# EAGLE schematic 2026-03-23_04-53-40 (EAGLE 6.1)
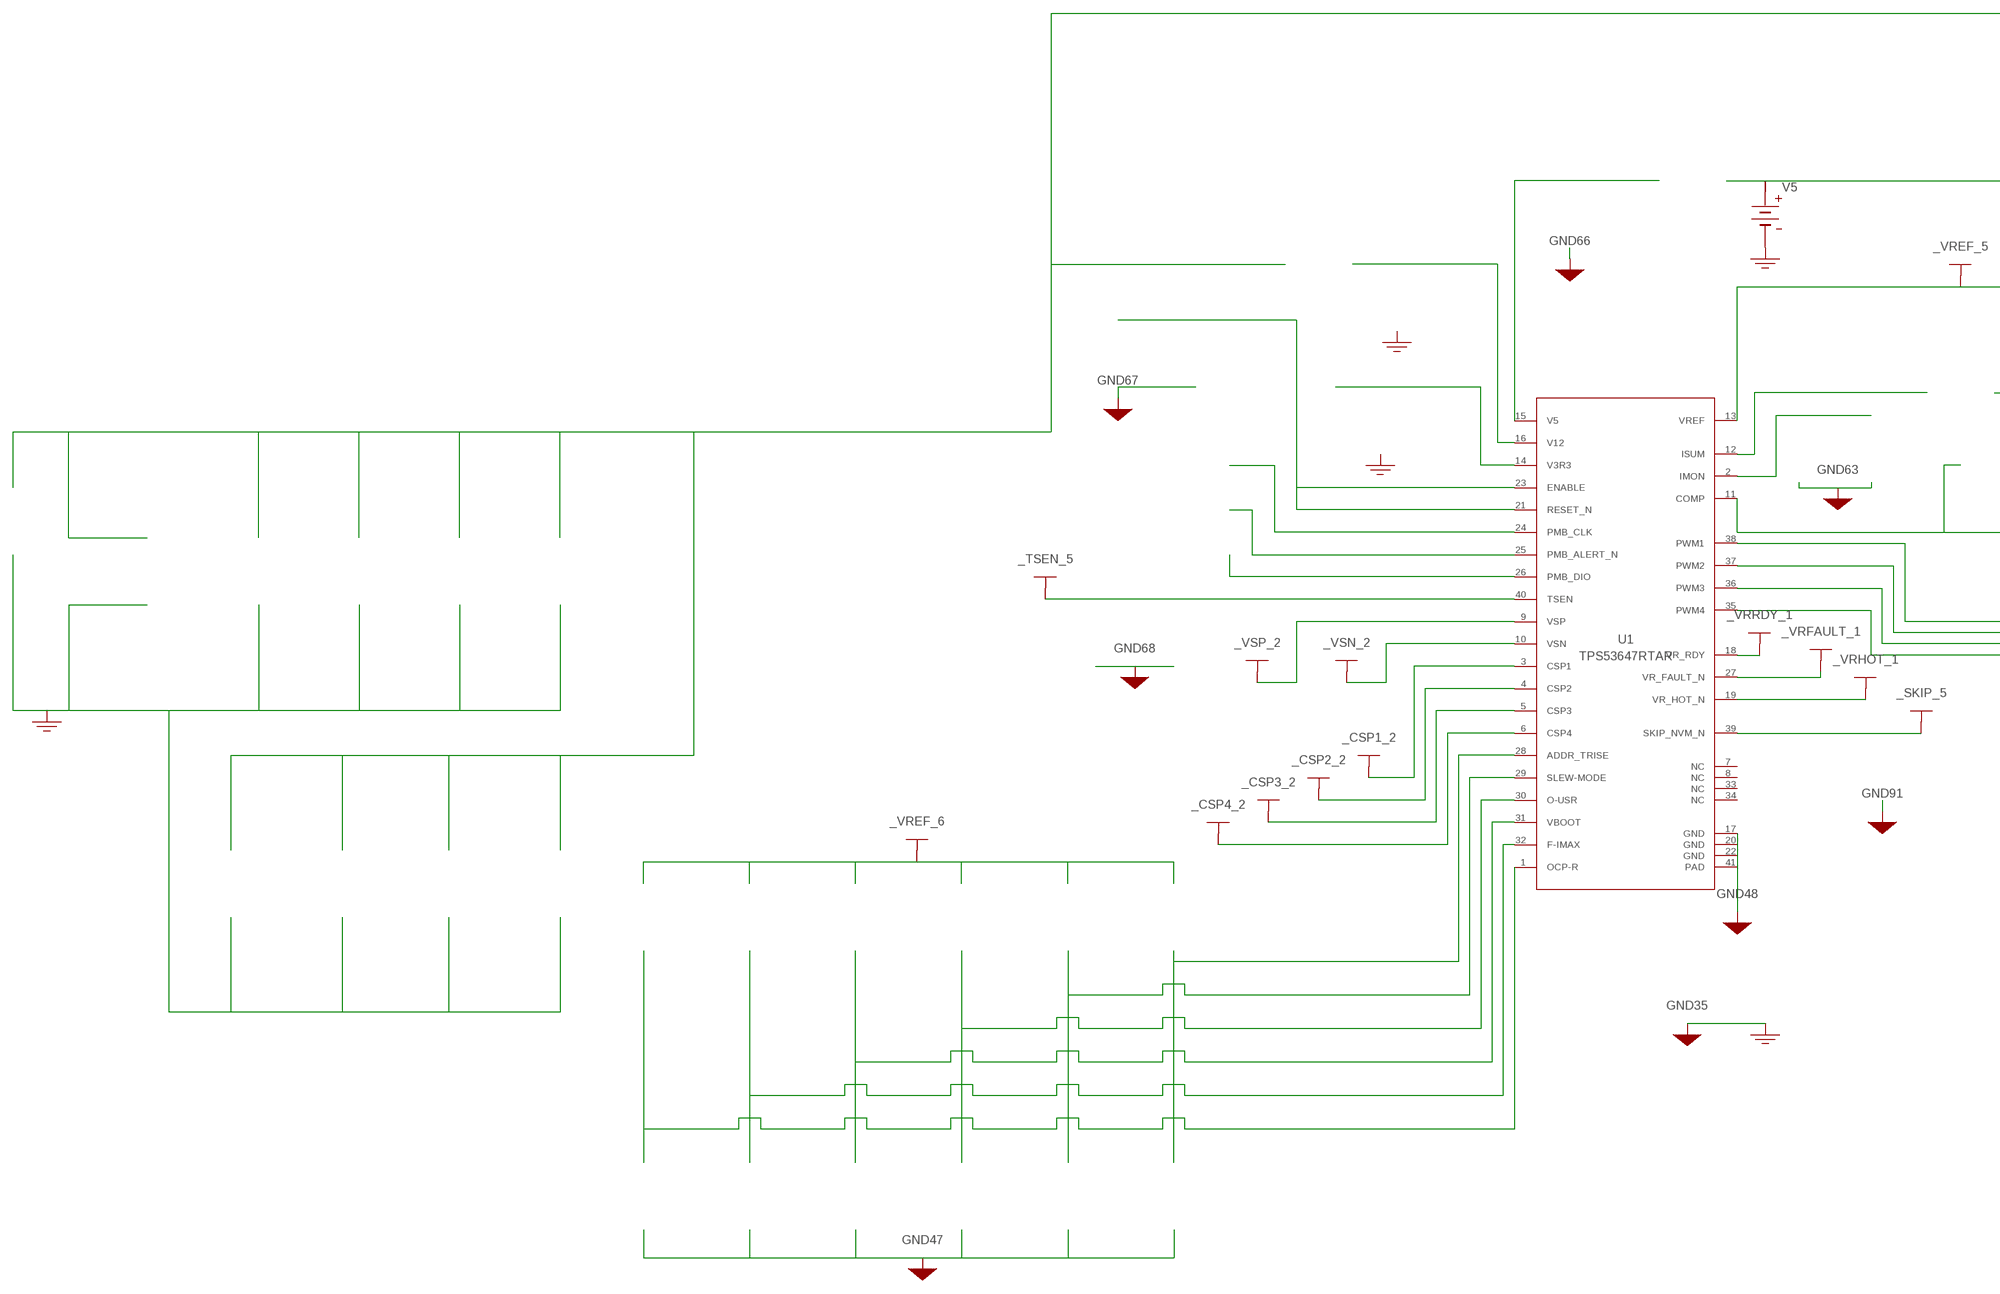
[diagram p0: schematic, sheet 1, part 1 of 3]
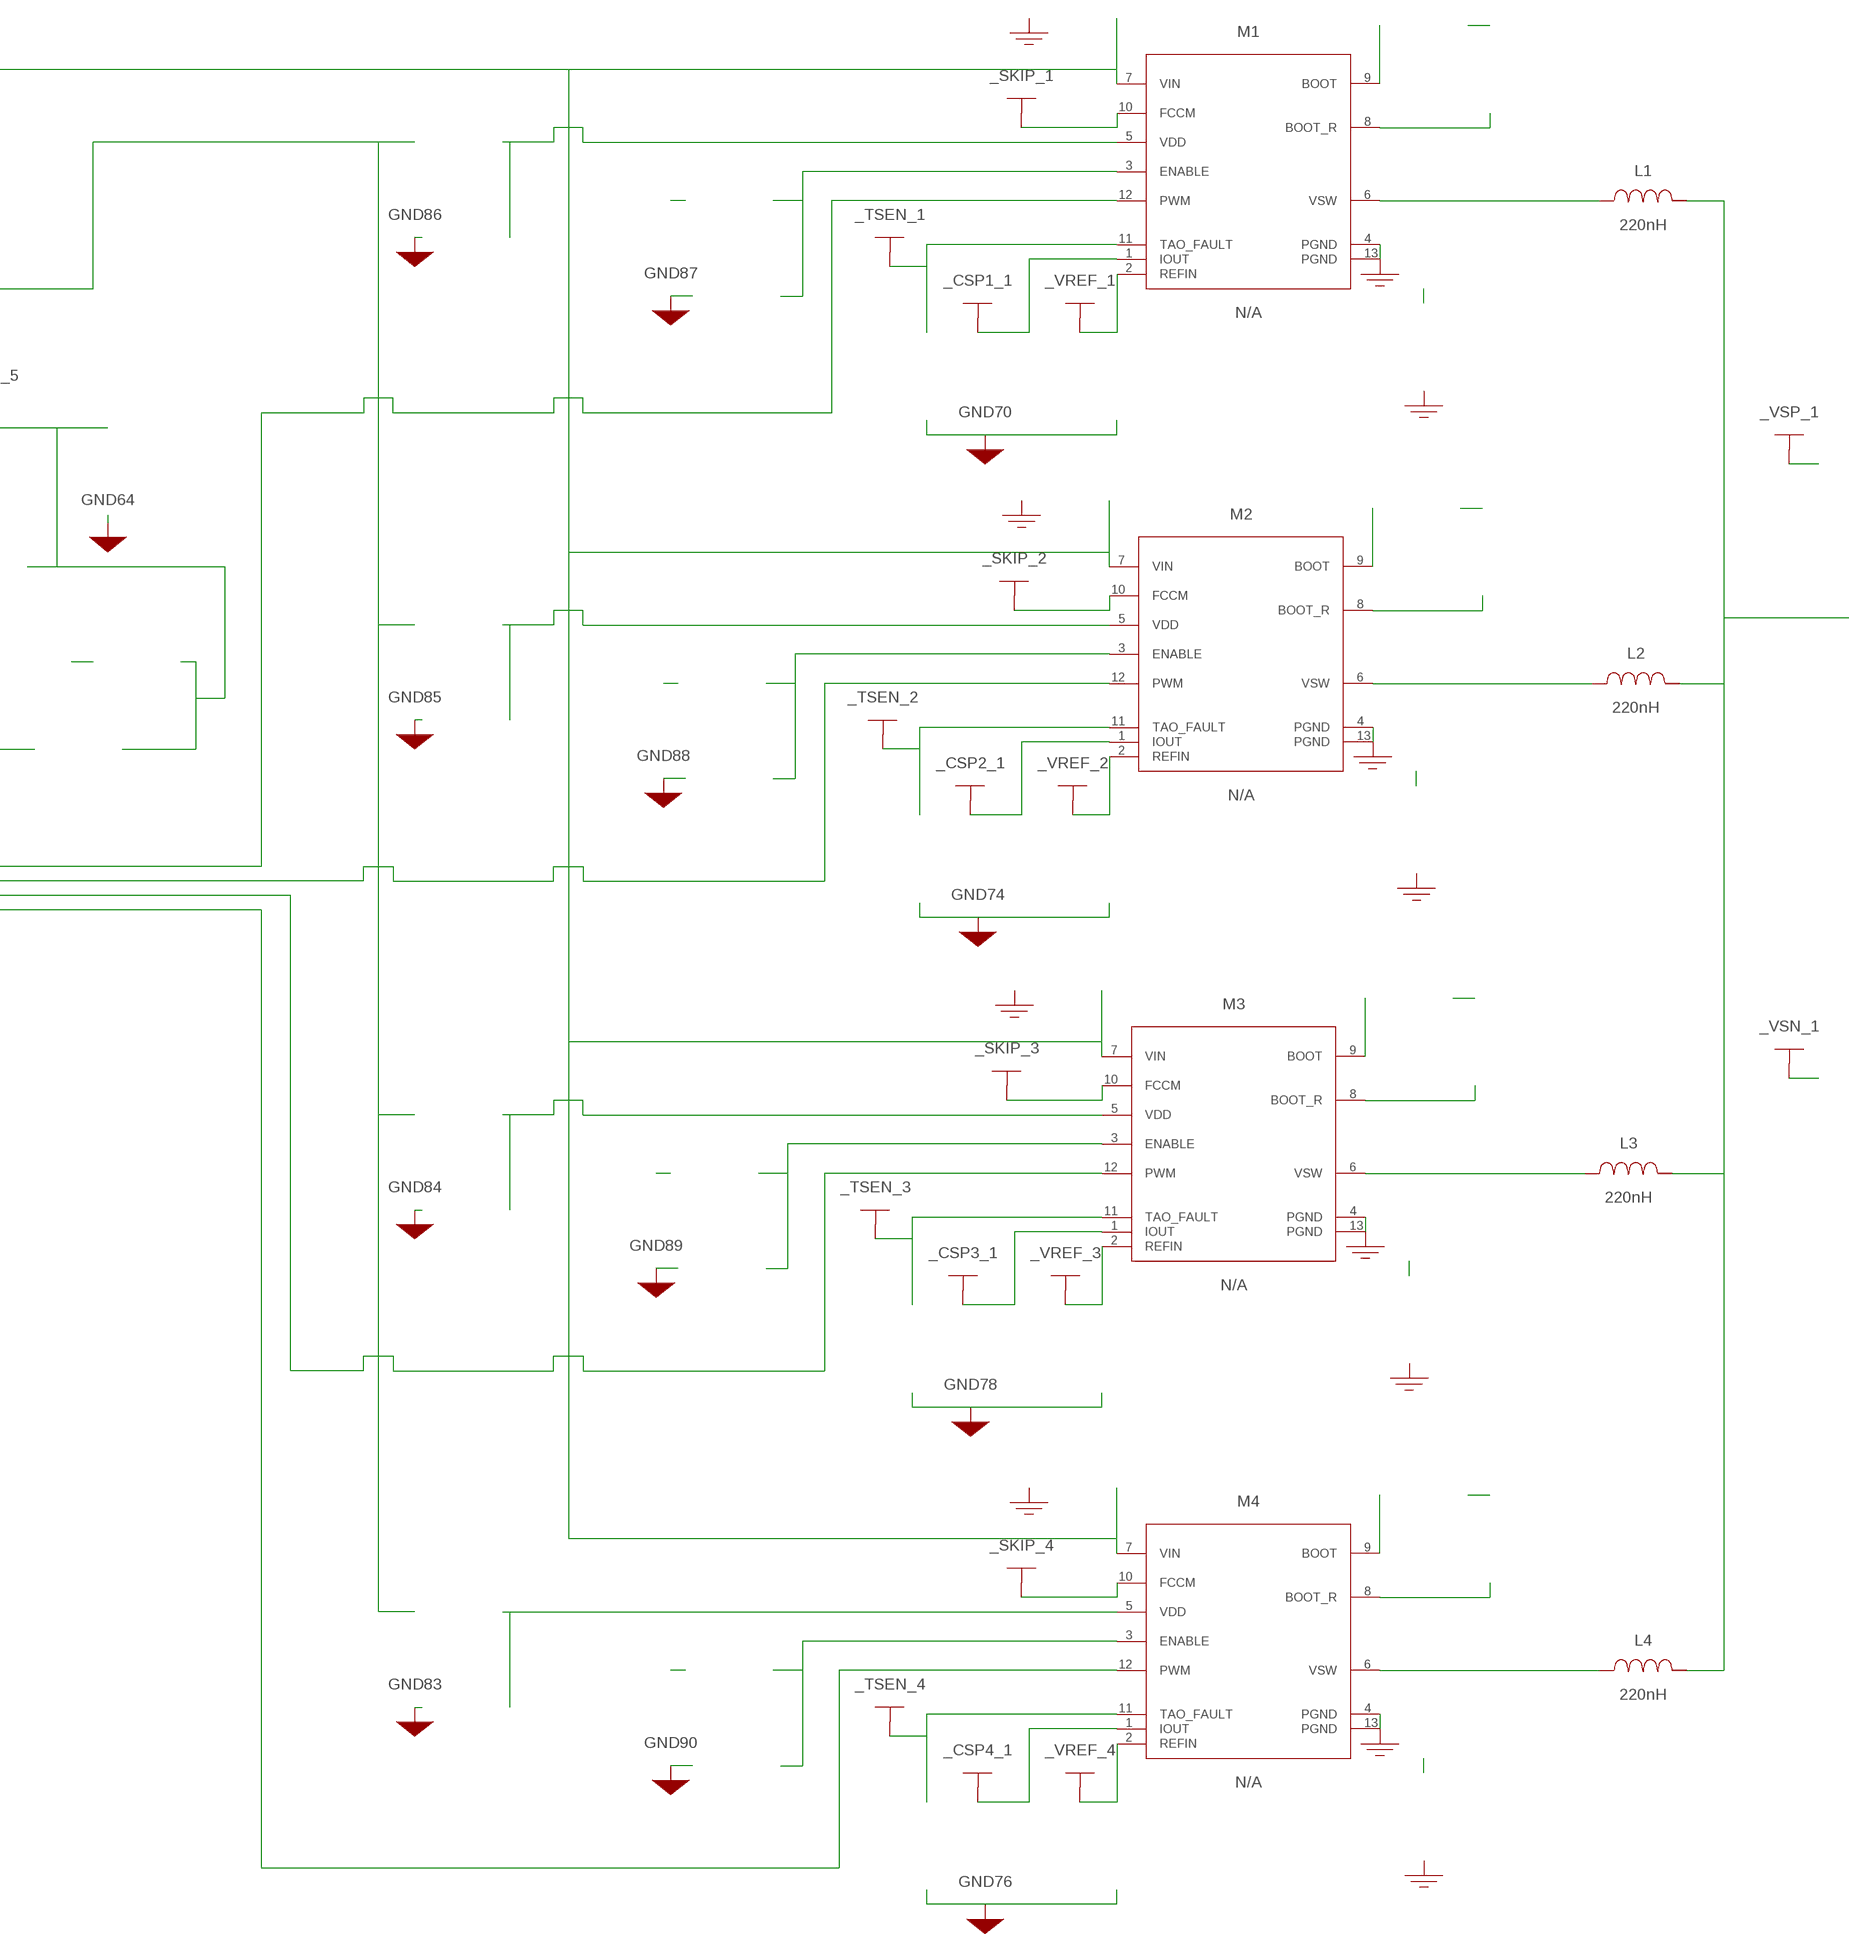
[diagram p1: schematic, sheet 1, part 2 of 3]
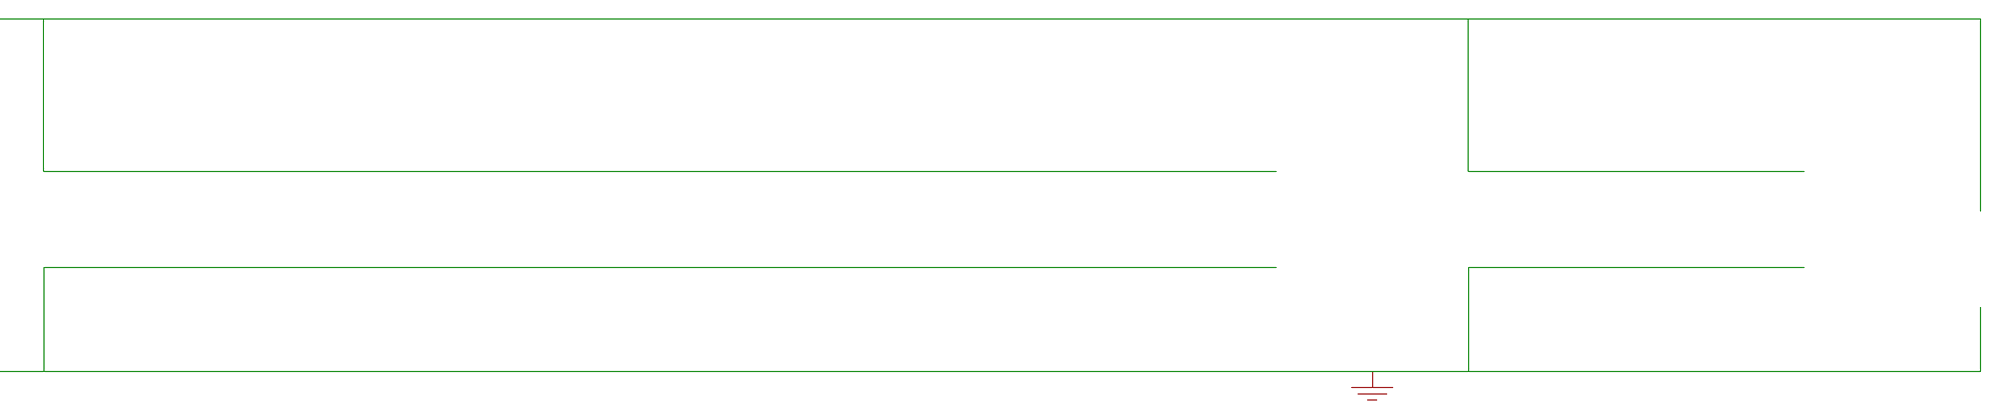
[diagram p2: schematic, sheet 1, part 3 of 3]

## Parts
_CSP1_1  WB_CONTINUATION  WB_CONTINUATIONWB_CONTINUATION  [WB_CONTINUATION]
_CSP1_2  WB_CONTINUATION  WB_CONTINUATIONWB_CONTINUATION  [WB_CONTINUATION]
_CSP2_1  WB_CONTINUATION  WB_CONTINUATIONWB_CONTINUATION  [WB_CONTINUATION]
_CSP2_2  WB_CONTINUATION  WB_CONTINUATIONWB_CONTINUATION  [WB_CONTINUATION]
_CSP3_1  WB_CONTINUATION  WB_CONTINUATIONWB_CONTINUATION  [WB_CONTINUATION]
_CSP3_2  WB_CONTINUATION  WB_CONTINUATIONWB_CONTINUATION  [WB_CONTINUATION]
_CSP4_1  WB_CONTINUATION  WB_CONTINUATIONWB_CONTINUATION  [WB_CONTINUATION]
_CSP4_2  WB_CONTINUATION  WB_CONTINUATIONWB_CONTINUATION  [WB_CONTINUATION]
_SKIP_1  WB_CONTINUATION  WB_CONTINUATIONWB_CONTINUATION  [WB_CONTINUATION]
_SKIP_2  WB_CONTINUATION  WB_CONTINUATIONWB_CONTINUATION  [WB_CONTINUATION]
_SKIP_3  WB_CONTINUATION  WB_CONTINUATIONWB_CONTINUATION  [WB_CONTINUATION]
_SKIP_4  WB_CONTINUATION  WB_CONTINUATIONWB_CONTINUATION  [WB_CONTINUATION]
_SKIP_5  WB_CONTINUATION  WB_CONTINUATIONWB_CONTINUATION  [WB_CONTINUATION]
_TSEN_1  WB_CONTINUATION  WB_CONTINUATIONWB_CONTINUATION  [WB_CONTINUATION]
_TSEN_2  WB_CONTINUATION  WB_CONTINUATIONWB_CONTINUATION  [WB_CONTINUATION]
_TSEN_3  WB_CONTINUATION  WB_CONTINUATIONWB_CONTINUATION  [WB_CONTINUATION]
_TSEN_4  WB_CONTINUATION  WB_CONTINUATIONWB_CONTINUATION  [WB_CONTINUATION]
_TSEN_5  WB_CONTINUATION  WB_CONTINUATIONWB_CONTINUATION  [WB_CONTINUATION]
_V3V3_1  WB_CONTINUATION  WB_CONTINUATIONWB_CONTINUATION  [WB_CONTINUATION]  (not placed on a sheet)
_V3V3_2  WB_CONTINUATION  WB_CONTINUATIONWB_CONTINUATION  [WB_CONTINUATION]  (not placed on a sheet)
_V3V3_3  WB_CONTINUATION  WB_CONTINUATIONWB_CONTINUATION  [WB_CONTINUATION]  (not placed on a sheet)
_V3V3_4  WB_CONTINUATION  WB_CONTINUATIONWB_CONTINUATION  [WB_CONTINUATION]  (not placed on a sheet)
_V3V3_5  WB_CONTINUATION  WB_CONTINUATIONWB_CONTINUATION  [WB_CONTINUATION]  (not placed on a sheet)
_VREF_1  WB_CONTINUATION  WB_CONTINUATIONWB_CONTINUATION  [WB_CONTINUATION]
_VREF_2  WB_CONTINUATION  WB_CONTINUATIONWB_CONTINUATION  [WB_CONTINUATION]
_VREF_3  WB_CONTINUATION  WB_CONTINUATIONWB_CONTINUATION  [WB_CONTINUATION]
_VREF_4  WB_CONTINUATION  WB_CONTINUATIONWB_CONTINUATION  [WB_CONTINUATION]
_VREF_5  WB_CONTINUATION  WB_CONTINUATIONWB_CONTINUATION  [WB_CONTINUATION]
_VREF_6  WB_CONTINUATION  WB_CONTINUATIONWB_CONTINUATION  [WB_CONTINUATION]
_VRFAULT_1  WB_CONTINUATION  WB_CONTINUATIONWB_CONTINUATION  [WB_CONTINUATION]
_VRHOT_1  WB_CONTINUATION  WB_CONTINUATIONWB_CONTINUATION  [WB_CONTINUATION]
_VRRDY_1  WB_CONTINUATION  WB_CONTINUATIONWB_CONTINUATION  [WB_CONTINUATION]
_VSN_1  WB_CONTINUATION  WB_CONTINUATIONWB_CONTINUATION  [WB_CONTINUATION]
_VSN_2  WB_CONTINUATION  WB_CONTINUATIONWB_CONTINUATION  [WB_CONTINUATION]
_VSP_1  WB_CONTINUATION  WB_CONTINUATIONWB_CONTINUATION  [WB_CONTINUATION]
_VSP_2  WB_CONTINUATION  WB_CONTINUATIONWB_CONTINUATION  [WB_CONTINUATION]
C3V3  1uF  C0603C105Z8VACTUC0603C105Z8VACTU  [0603]  (not placed on a sheet)
CBP3  1uF  C0603C105Z8VACTUC0603C105Z8VACTU  [0603]  (not placed on a sheet)
CBST1  100nF  EMK107B7104KA-TEMK107B7104KA-T  [0603]  (not placed on a sheet)
CBST2  100nF  EMK107B7104KA-TEMK107B7104KA-T  [0603]  (not placed on a sheet)
CBST3  100nF  EMK107B7104KA-TEMK107B7104KA-T  [0603]  (not placed on a sheet)
CBST4  100nF  EMK107B7104KA-TEMK107B7104KA-T  [0603]  (not placed on a sheet)
CCOMP  1nF  GRM1555C1H102JA01JGRM1555C1H102JA01J  [0402]  (not placed on a sheet)
CCOMP2  22pF  CL21C220JBANNNCCL21C220JBANNNC  [0805]  (not placed on a sheet)
CDD  1uF  C1608X5R1E105K080ACC1608X5R1E105K080AC  [0603]  (not placed on a sheet)
CEN1  1nF  CC0603JRNPO8BN102CC0603JRNPO8BN102  [0603]  (not placed on a sheet)
CEN2  1nF  CC0603JRNPO8BN102CC0603JRNPO8BN102  [0603]  (not placed on a sheet)
CEN3  1nF  CC0603JRNPO8BN102CC0603JRNPO8BN102  [0603]  (not placed on a sheet)
CEN4  1nF  CC0603JRNPO8BN102CC0603JRNPO8BN102  [0603]  (not placed on a sheet)
CHF1  3.3nF  CGA1A2X7R1E332K030BACGA1A2X7R1E332K030BA  [0201_033]  (not placed on a sheet)
CHF2  3.3nF  CGA1A2X7R1E332K030BACGA1A2X7R1E332K030BA  [0201_033]  (not placed on a sheet)
CHF3  3.3nF  CGA1A2X7R1E332K030BACGA1A2X7R1E332K030BA  [0201_033]  (not placed on a sheet)
CHF4  3.3nF  CGA1A2X7R1E332K030BACGA1A2X7R1E332K030BA  [0201_033]  (not placed on a sheet)
CIMON  2.2nF  GRM033R71A222KA01DGRM033R71A222KA01D  [0201]  (not placed on a sheet)
CIN  270uF  16SVPG270M16SVPG270M  [CAPSMT_62_C10]  (not placed on a sheet)
CIN_2  270uF  16SVPG270M16SVPG270M  [CAPSMT_62_C10]  (not placed on a sheet)
CINX_CH1  22uF  MSASE21GBB5226MTNA01MSASE21GBB5226MTNA01  [0805]  (not placed on a sheet)
CINX_CH2  22uF  MSASE21GBB5226MTNA01MSASE21GBB5226MTNA01  [0805]  (not placed on a sheet)
CINX_CH3  22uF  MSASE21GBB5226MTNA01MSASE21GBB5226MTNA01  [0805]  (not placed on a sheet)
CINX_CH4  22uF  MSASE21GBB5226MTNA01MSASE21GBB5226MTNA01  [0805]  (not placed on a sheet)
CINX_CH5  47uF  GRM32ER61C476KE15LGRM32ER61C476KE15L  [1210_280]  (not placed on a sheet)
CINX_CH6  47uF  GRM32ER61C476KE15LGRM32ER61C476KE15L  [1210_280]  (not placed on a sheet)
CINX_CH7  47uF  GRM32ER61C476KE15LGRM32ER61C476KE15L  [1210_280]  (not placed on a sheet)
CINX_CH8  47uF  GRM32ER61C476KE15LGRM32ER61C476KE15L  [1210_280]  (not placed on a sheet)
COUT  470uF  EEFGX0D471REEFGX0D471R  [7343-20]  (not placed on a sheet)
COUT_2  470uF  EEFGX0D471REEFGX0D471R  [7343-20]  (not placed on a sheet)
COUT_3  470uF  EEFGX0D471REEFGX0D471R  [7343-20]  (not placed on a sheet)
COUT_4  470uF  EEFGX0D471REEFGX0D471R  [7343-20]  (not placed on a sheet)
COUTX_CH1  100uF  GRM32EC80J107ME20LGRM32EC80J107ME20L  [1210_270]  (not placed on a sheet)
COUTX_CH1_2  100uF  GRM32EC80J107ME20LGRM32EC80J107ME20L  [1210_270]  (not placed on a sheet)
COUTX_CH1_3  100uF  GRM32EC80J107ME20LGRM32EC80J107ME20L  [1210_270]  (not placed on a sheet)
COUTX_CH1_4  100uF  GRM32EC80J107ME20LGRM32EC80J107ME20L  [1210_270]  (not placed on a sheet)
COUTX_CH1_5  100uF  GRM32EC80J107ME20LGRM32EC80J107ME20L  [1210_270]  (not placed on a sheet)
COUTX_CH1_6  100uF  GRM32EC80J107ME20LGRM32EC80J107ME20L  [1210_270]  (not placed on a sheet)
COUTX_CH1_7  100uF  GRM32EC80J107ME20LGRM32EC80J107ME20L  [1210_270]  (not placed on a sheet)
COUTX_CH1_8  100uF  GRM32EC80J107ME20LGRM32EC80J107ME20L  [1210_270]  (not placed on a sheet)
COUTX_CH1_9  100uF  GRM32EC80J107ME20LGRM32EC80J107ME20L  [1210_270]  (not placed on a sheet)
COUTX_CH1_10  100uF  GRM32EC80J107ME20LGRM32EC80J107ME20L  [1210_270]  (not placed on a sheet)
COUTX_CH1_11  100uF  GRM32EC80J107ME20LGRM32EC80J107ME20L  [1210_270]  (not placed on a sheet)
COUTX_CH1_12  100uF  GRM32EC80J107ME20LGRM32EC80J107ME20L  [1210_270]  (not placed on a sheet)
COUTX_CH2  100uF  GRM32EC80J107ME20LGRM32EC80J107ME20L  [1210_270]  (not placed on a sheet)
COUTX_CH2_2  100uF  GRM32EC80J107ME20LGRM32EC80J107ME20L  [1210_270]  (not placed on a sheet)
COUTX_CH2_3  100uF  GRM32EC80J107ME20LGRM32EC80J107ME20L  [1210_270]  (not placed on a sheet)
COUTX_CH2_4  100uF  GRM32EC80J107ME20LGRM32EC80J107ME20L  [1210_270]  (not placed on a sheet)
COUTX_CH2_5  100uF  GRM32EC80J107ME20LGRM32EC80J107ME20L  [1210_270]  (not placed on a sheet)
COUTX_CH2_6  100uF  GRM32EC80J107ME20LGRM32EC80J107ME20L  [1210_270]  (not placed on a sheet)
COUTX_CH2_7  100uF  GRM32EC80J107ME20LGRM32EC80J107ME20L  [1210_270]  (not placed on a sheet)
COUTX_CH2_8  100uF  GRM32EC80J107ME20LGRM32EC80J107ME20L  [1210_270]  (not placed on a sheet)
COUTX_CH2_9  100uF  GRM32EC80J107ME20LGRM32EC80J107ME20L  [1210_270]  (not placed on a sheet)
COUTX_CH2_10  100uF  GRM32EC80J107ME20LGRM32EC80J107ME20L  [1210_270]  (not placed on a sheet)
COUTX_CH2_11  100uF  GRM32EC80J107ME20LGRM32EC80J107ME20L  [1210_270]  (not placed on a sheet)
COUTX_CH2_12  100uF  GRM32EC80J107ME20LGRM32EC80J107ME20L  [1210_270]  (not placed on a sheet)
CREF  330nF  C0603C334K8RACTUC0603C334K8RACTU  [0603]  (not placed on a sheet)
CREF1  100nF  08053C104KAT2A08053C104KAT2A  [0805]  (not placed on a sheet)
CREF2  100nF  08053C104KAT2A08053C104KAT2A  [0805]  (not placed on a sheet)
CREF3  100nF  08053C104KAT2A08053C104KAT2A  [0805]  (not placed on a sheet)
CREF4  100nF  08053C104KAT2A08053C104KAT2A  [0805]  (not placed on a sheet)
CSNUB1  1nF  CC0603JRNPO8BN102CC0603JRNPO8BN102  [0603]  (not placed on a sheet)
CSNUB2  1nF  CC0603JRNPO8BN102CC0603JRNPO8BN102  [0603]  (not placed on a sheet)
CSNUB3  1nF  CC0603JRNPO8BN102CC0603JRNPO8BN102  [0603]  (not placed on a sheet)
CSNUB4  1nF  CC0603JRNPO8BN102CC0603JRNPO8BN102  [0603]  (not placed on a sheet)
CTAO1  1nF  GRM033R71C102KA01DGRM033R71C102KA01D  [0201]  (not placed on a sheet)
CTAO2  1nF  GRM033R71C102KA01DGRM033R71C102KA01D  [0201]  (not placed on a sheet)
CTAO3  1nF  GRM033R71C102KA01DGRM033R71C102KA01D  [0201]  (not placed on a sheet)
CTAO4  1nF  GRM033R71C102KA01DGRM033R71C102KA01D  [0201]  (not placed on a sheet)
CTSEN  1nF  GRM033R71C102KA01DGRM033R71C102KA01D  [0201]  (not placed on a sheet)
CV5  4.7uF  C1608X5R1C475K080ACC1608X5R1C475K080AC  [0603]  (not placed on a sheet)
CVDD1  2.2uF  EMK212BJ225KG-TEMK212BJ225KG-T  [0805]  (not placed on a sheet)
CVDD2  2.2uF  EMK212BJ225KG-TEMK212BJ225KG-T  [0805]  (not placed on a sheet)
CVDD3  2.2uF  EMK212BJ225KG-TEMK212BJ225KG-T  [0805]  (not placed on a sheet)
CVDD4  2.2uF  EMK212BJ225KG-TEMK212BJ225KG-T  [0805]  (not placed on a sheet)
GND10  WB_GND  WB_GNDWB_GND  [WB_GND]
GND14  WB_GND  WB_GNDWB_GND  [WB_GND]
GND17  WB_GND  WB_GNDWB_GND  [WB_GND]
GND18  WB_GND  WB_GNDWB_GND  [WB_GND]
GND29  WB_GND  WB_GNDWB_GND  [WB_GND]
GND34  WB_GND  WB_GNDWB_GND  [WB_GND]
GND35  WB_GND_SIGNAL  WB_GND_SIGNALWB_GND_SIGNAL  [WB_GND_SIGNAL]
GND36  WB_GND  WB_GNDWB_GND  [WB_GND]
GND38  WB_GND  WB_GNDWB_GND  [WB_GND]
GND40  WB_GND  WB_GNDWB_GND  [WB_GND]
GND42  WB_GND  WB_GNDWB_GND  [WB_GND]
GND44  WB_GND  WB_GNDWB_GND  [WB_GND]
GND46  WB_GND  WB_GNDWB_GND  [WB_GND]
GND47  WB_GND_SIGNAL  WB_GND_SIGNALWB_GND_SIGNAL  [WB_GND_SIGNAL]
GND48  WB_GND_SIGNAL  WB_GND_SIGNALWB_GND_SIGNAL  [WB_GND_SIGNAL]
GND49  WB_GND  WB_GNDWB_GND  [WB_GND]
GND62  WB_GND  WB_GNDWB_GND  [WB_GND]
GND63  WB_GND_SIGNAL  WB_GND_SIGNALWB_GND_SIGNAL  [WB_GND_SIGNAL]
GND64  WB_GND_SIGNAL  WB_GND_SIGNALWB_GND_SIGNAL  [WB_GND_SIGNAL]
GND66  WB_GND_SIGNAL  WB_GND_SIGNALWB_GND_SIGNAL  [WB_GND_SIGNAL]
GND67  WB_GND_SIGNAL  WB_GND_SIGNALWB_GND_SIGNAL  [WB_GND_SIGNAL]
GND68  WB_GND_SIGNAL  WB_GND_SIGNALWB_GND_SIGNAL  [WB_GND_SIGNAL]
GND70  WB_GND_SIGNAL  WB_GND_SIGNALWB_GND_SIGNAL  [WB_GND_SIGNAL]
GND72  WB_GND  WB_GNDWB_GND  [WB_GND]
GND73  WB_GND  WB_GNDWB_GND  [WB_GND]
GND74  WB_GND_SIGNAL  WB_GND_SIGNALWB_GND_SIGNAL  [WB_GND_SIGNAL]
GND75  WB_GND  WB_GNDWB_GND  [WB_GND]
GND76  WB_GND_SIGNAL  WB_GND_SIGNALWB_GND_SIGNAL  [WB_GND_SIGNAL]
GND77  WB_GND  WB_GNDWB_GND  [WB_GND]
GND78  WB_GND_SIGNAL  WB_GND_SIGNALWB_GND_SIGNAL  [WB_GND_SIGNAL]
GND79  WB_GND  WB_GNDWB_GND  [WB_GND]
GND83  WB_GND_SIGNAL  WB_GND_SIGNALWB_GND_SIGNAL  [WB_GND_SIGNAL]
GND84  WB_GND_SIGNAL  WB_GND_SIGNALWB_GND_SIGNAL  [WB_GND_SIGNAL]
GND85  WB_GND_SIGNAL  WB_GND_SIGNALWB_GND_SIGNAL  [WB_GND_SIGNAL]
GND86  WB_GND_SIGNAL  WB_GND_SIGNALWB_GND_SIGNAL  [WB_GND_SIGNAL]
GND87  WB_GND_SIGNAL  WB_GND_SIGNALWB_GND_SIGNAL  [WB_GND_SIGNAL]
GND88  WB_GND_SIGNAL  WB_GND_SIGNALWB_GND_SIGNAL  [WB_GND_SIGNAL]
GND89  WB_GND_SIGNAL  WB_GND_SIGNALWB_GND_SIGNAL  [WB_GND_SIGNAL]
GND90  WB_GND_SIGNAL  WB_GND_SIGNALWB_GND_SIGNAL  [WB_GND_SIGNAL]
GND91  WB_GND_SIGNAL  WB_GND_SIGNALWB_GND_SIGNAL  [WB_GND_SIGNAL]
L1  220nH  74430820227443082022  [WE-HCM_1088]
L2  220nH  74430820227443082022  [WE-HCM_1088]
L3  220nH  74430820227443082022  [WE-HCM_1088]
L4  220nH  74430820227443082022  [WE-HCM_1088]
M1  N/A  CSD95372BQ5MCSD95372BQ5M  [DQP0012A]
M2  N/A  CSD95372BQ5MCSD95372BQ5M  [DQP0012A]
M3  N/A  CSD95372BQ5MCSD95372BQ5M  [DQP0012A]
M4  N/A  CSD95372BQ5MCSD95372BQ5M  [DQP0012A]
RADDR  16.5k  CRCW040216K5FKEDCRCW040216K5FKED  [0402]  (not placed on a sheet)
RBST1  1  CRCW04021R00FKEDCRCW04021R00FKED  [0402]  (not placed on a sheet)
RBST2  1  CRCW04021R00FKEDCRCW04021R00FKED  [0402]  (not placed on a sheet)
RBST3  1  CRCW04021R00FKEDCRCW04021R00FKED  [0402]  (not placed on a sheet)
RBST4  1  CRCW04021R00FKEDCRCW04021R00FKED  [0402]  (not placed on a sheet)
RCOMP  3.83k  CRCW04023K83FKEDCRCW04023K83FKED  [0402]  (not placed on a sheet)
RDD  1  CRCW04021R00FKEDCRCW04021R00FKED  [0402]  (not placed on a sheet)
REN1  10k  RC0201FR-0710KLRC0201FR-0710KL  [0201]  (not placed on a sheet)
REN2  10k  RC0201FR-0710KLRC0201FR-0710KL  [0201]  (not placed on a sheet)
REN3  10k  RC0201FR-0710KLRC0201FR-0710KL  [0201]  (not placed on a sheet)
REN4  10k  RC0201FR-0710KLRC0201FR-0710KL  [0201]  (not placed on a sheet)
RF  23.7k  RC0201FR-0723K7LRC0201FR-0723K7L  [0201]  (not placed on a sheet)
RIMAX  26.1k  CRCW040226K1FKEDCRCW040226K1FKED  [0402]  (not placed on a sheet)
RIMON  49.9k  CRCW040249K9FKEDCRCW040249K9FKED  [0402]  (not placed on a sheet)
RISUM  2.55k  CRCW04022K55FKEDCRCW04022K55FKED  [0402]  (not placed on a sheet)
RLOAD  WB_LOAD_RESISTOR  WB_LOAD_RESISTORWB_LOAD_RESISTOR  [WB_LOAD_RESISTOR]  (not placed on a sheet)
RMODE  16.5k  CRCW040216K5FKEDCRCW040216K5FKED  [0402]  (not placed on a sheet)
RNVM  20k  CRCW040220K0FKEDCRCW040220K0FKED  [0402]  (not placed on a sheet)
ROCPR  20k  CRCW040220K0FKEDCRCW040220K0FKED  [0402]  (not placed on a sheet)
ROSR  150k  CRCW0402150KFKEDCRCW0402150KFKED  [0402]  (not placed on a sheet)
RRAMP  4.32k  CRCW04024K32FKEDCRCW04024K32FKED  [0402]  (not placed on a sheet)
RSLEW  24.3k  CRCW040224K3FKEDCRCW040224K3FKED  [0402]  (not placed on a sheet)
RSN  1  CRCW04021R00FKEDCRCW04021R00FKED  [0402]  (not placed on a sheet)
RSNUB1  1  CRCW04021R00FKEDCRCW04021R00FKED  [0402]  (not placed on a sheet)
RSNUB2  1  CRCW04021R00FKEDCRCW04021R00FKED  [0402]  (not placed on a sheet)
RSNUB3  1  CRCW04021R00FKEDCRCW04021R00FKED  [0402]  (not placed on a sheet)
RSNUB4  1  CRCW04021R00FKEDCRCW04021R00FKED  [0402]  (not placed on a sheet)
RSP  1  CRCW04021R00FKEDCRCW04021R00FKED  [0402]  (not placed on a sheet)
RTRISE  24.3k  CRCW040224K3FKEDCRCW040224K3FKED  [0402]  (not placed on a sheet)
RTSEN  121k  CRCW0402121KFKEDCRCW0402121KFKED  [0402]  (not placed on a sheet)
RUSR  9.31k  CRCW04029K31FKEDCRCW04029K31FKED  [0402]  (not placed on a sheet)
RV5  1  CRCW04021R00FKEDCRCW04021R00FKED  [0402]  (not placed on a sheet)
RVBOOTB  39.2k  CRCW040239K2FKEDCRCW040239K2FKED  [0402]  (not placed on a sheet)
RVBOOTT  26.7k  CRCW040226K7FKEDCRCW040226K7FKED  [0402]  (not placed on a sheet)
RVDD1  1  CRCW04021R00FKEDCRCW04021R00FKED  [0402]  (not placed on a sheet)
RVDD2  1  CRCW04021R00FKEDCRCW04021R00FKED  [0402]  (not placed on a sheet)
RVDD3  1  CRCW04021R00FKEDCRCW04021R00FKED  [0402]  (not placed on a sheet)
RVDD4  1  CRCW04021R00FKEDCRCW04021R00FKED  [0402]  (not placed on a sheet)
U1  TPS53647RTAR  TPS53647RTARTPS53647RTAR  [RTA0040B]
V3V3  WB_PRIMITIVE_BATTERY  WB_PRIMITIVE_BATTERYWB_PRIMITIVE_BATTERY  [WB_PRIMITIVE_BATTERY]  (not placed on a sheet)
V5  WB_PRIMITIVE_BATTERY  WB_PRIMITIVE_BATTERYWB_PRIMITIVE_BATTERY  [WB_PRIMITIVE_BATTERY]
VALERT  WB_PMBUS_ALERT  WB_PMBUS_ALERTWB_PMBUS_ALERT  [WB_PMBUS_ALERT]  (not placed on a sheet)
VIN  WB_BATTERY  WB_BATTERYWB_BATTERY  [WB_BATTERY]  (not placed on a sheet)
VSCL  WB_I2C_SCL  WB_I2C_SCLWB_I2C_SCL  [WB_I2C_SCL]  (not placed on a sheet)
VSDA  WB_I2C_SDA  WB_I2C_SDAWB_I2C_SDA  [WB_I2C_SDA]  (not placed on a sheet)
Unconnected: _CSP1_1.1(Node) _CSP1_2.1(Node) _CSP2_1.1(Node) _CSP2_2.1(Node) _CSP3_1.1(Node) _CSP3_2.1(Node) _CSP4_1.1(Node) _CSP4_2.1(Node) _SKIP_1.1(Node) _SKIP_2.1(Node) _SKIP_3.1(Node) _SKIP_4.1(Node) _SKIP_5.1(Node) _TSEN_1.1(Node) _TSEN_2.1(Node) _TSEN_3.1(Node) _TSEN_4.1(Node) _TSEN_5.1(Node) _V3V3_1.1(Node) _V3V3_2.1(Node) _V3V3_3.1(Node) _V3V3_4.1(Node) _V3V3_5.1(Node) _VREF_1.1(Node) _VREF_2.1(Node) _VREF_3.1(Node) _VREF_4.1(Node) _VREF_5.1(Node) _VREF_6.1(Node) _VRFAULT_1.1(Node) _VRHOT_1.1(Node) _VRRDY_1.1(Node) _VSN_1.1(Node) _VSN_2.1(Node) _VSP_1.1(Node) _VSP_2.1(Node) C3V3.1 C3V3.2 CBP3.1 CBP3.2 CBST1.1 CBST1.2 CBST2.1 CBST2.2 CBST3.1 CBST3.2 CBST4.1 CBST4.2 CCOMP2.1 CCOMP2.2 CCOMP.1 CCOMP.2 CDD.1 CDD.2 CEN1.1 CEN1.2 CEN2.1 CEN2.2 CEN3.1 CEN3.2 CEN4.1 CEN4.2 CHF1.1 CHF1.2 CHF2.1 CHF2.2 CHF3.1 CHF3.2 CHF4.1 CHF4.2 CIMON.1 CIMON.2 CIN.1(+) CIN.2(-) CIN_2.1(+) CIN_2.2(-) CINX_CH1.1 CINX_CH1.2 CINX_CH2.1 CINX_CH2.2 CINX_CH3.1 CINX_CH3.2 CINX_CH4.1 CINX_CH4.2 CINX_CH5.1 CINX_CH5.2 CINX_CH6.1 CINX_CH6.2 CINX_CH7.1 CINX_CH7.2 CINX_CH8.1 CINX_CH8.2 COUT.1(+) COUT.2(-) COUT_2.1(+) COUT_2.2(-) COUT_3.1(+) COUT_3.2(-) COUT_4.1(+) COUT_4.2(-) COUTX_CH1.1 COUTX_CH1.2 COUTX_CH1_2.1 COUTX_CH1_2.2 COUTX_CH1_3.1 COUTX_CH1_3.2 COUTX_CH1_4.1 COUTX_CH1_4.2 COUTX_CH1_5.1 COUTX_CH1_5.2 COUTX_CH1_6.1 COUTX_CH1_6.2 COUTX_CH1_7.1 COUTX_CH1_7.2 COUTX_CH1_8.1 COUTX_CH1_8.2 COUTX_CH1_9.1 COUTX_CH1_9.2 COUTX_CH1_10.1 COUTX_CH1_10.2 COUTX_CH1_11.1 COUTX_CH1_11.2 COUTX_CH1_12.1 COUTX_CH1_12.2 COUTX_CH2.1 COUTX_CH2.2 COUTX_CH2_2.1 COUTX_CH2_2.2 COUTX_CH2_3.1 COUTX_CH2_3.2 COUTX_CH2_4.1 COUTX_CH2_4.2 COUTX_CH2_5.1 COUTX_CH2_5.2 COUTX_CH2_6.1 COUTX_CH2_6.2 COUTX_CH2_7.1 COUTX_CH2_7.2 COUTX_CH2_8.1 COUTX_CH2_8.2 COUTX_CH2_9.1 COUTX_CH2_9.2 COUTX_CH2_10.1 COUTX_CH2_10.2 COUTX_CH2_11.1 COUTX_CH2_11.2 COUTX_CH2_12.1 COUTX_CH2_12.2 CREF1.1 CREF1.2 CREF2.1 CREF2.2 CREF3.1 CREF3.2 CREF4.1 CREF4.2 CREF.1 CREF.2 CSNUB1.1 CSNUB1.2 CSNUB2.1 CSNUB2.2 CSNUB3.1 CSNUB3.2 CSNUB4.1 CSNUB4.2 CTAO1.1 CTAO1.2 CTAO2.1 CTAO2.2 CTAO3.1 CTAO3.2 CTAO4.1 CTAO4.2 CTSEN.1 CTSEN.2 CV5.1 CV5.2 CVDD1.1 CVDD1.2 CVDD2.1 CVDD2.2 CVDD3.1 CVDD3.2 CVDD4.1 CVDD4.2 GND10.1 GND14.1 GND17.1 GND18.1 GND29.1 GND34.1 GND35.1 GND36.1 GND38.1 GND40.1 GND42.1 GND44.1 GND46.1 GND47.1 GND48.1 GND49.1 GND62.1 GND63.1 GND64.1 GND66.1 GND67.1 GND68.1 GND70.1 GND72.1 GND73.1 GND74.1 GND75.1 GND76.1 GND77.1 GND78.1 GND79.1 GND83.1 GND84.1 GND85.1 GND86.1 GND87.1 GND88.1 GND89.1 GND90.1 GND91.1 L1.1 L1.2 L2.1 L2.2 L3.1 L3.2 L4.1 L4.2 M1.1(IOUT) M1.2(REFIN) M1.3(ENABLE) M1.9(BOOT) M1.10(FCCM) M1.11(TAO_FAULT) M1.12(PWM) M2.1(IOUT) M2.2(REFIN) M2.3(ENABLE) M2.9(BOOT) M2.10(FCCM) M2.11(TAO_FAULT) M2.12(PWM) M3.1(IOUT) M3.2(REFIN) M3.3(ENABLE) M3.9(BOOT) M3.10(FCCM) M3.11(TAO_FAULT) M3.12(PWM) M4.1(IOUT) M4.2(REFIN) M4.3(ENABLE) M4.9(BOOT) M4.10(FCCM) M4.11(TAO_FAULT) M4.12(PWM) RADDR.1 RADDR.2 RBST1.1 RBST1.2 RBST2.1 RBST2.2 RBST3.1 RBST3.2 RBST4.1 RBST4.2 RCOMP.1 RCOMP.2 RDD.1 RDD.2 REN1.1 REN1.2 REN2.1 REN2.2 REN3.1 REN3.2 REN4.1 REN4.2 RF.1 RF.2 RIMAX.1 RIMAX.2 RIMON.1 RIMON.2 RISUM.1 RISUM.2 RLOAD.1 RLOAD.2 RMODE.1 RMODE.2 RNVM.1 RNVM.2 ROCPR.1 ROCPR.2 ROSR.1 ROSR.2 RRAMP.1 RRAMP.2 RSLEW.1 RSLEW.2 RSN.1 RSN.2 RSNUB1.1 RSNUB1.2 RSNUB2.1 RSNUB2.2 RSNUB3.1 RSNUB3.2 RSNUB4.1 RSNUB4.2 RSP.1 RSP.2 RTRISE.1 RTRISE.2 RTSEN.1 RTSEN.2 RUSR.1 RUSR.2 RV5.1 RV5.2 RVBOOTB.1 RVBOOTB.2 RVBOOTT.1 RVBOOTT.2 RVDD1.1 RVDD1.2 RVDD2.1 RVDD2.2 RVDD3.1 RVDD3.2 RVDD4.1 RVDD4.2 U1.1(OCP-R) U1.2(IMON) U1.3(CSP1) U1.4(CSP2) U1.5(CSP3) U1.6(CSP4) U1.7(NC) U1.8(NC) U1.9(VSP) U1.10(VSN) U1.11(COMP) U1.12(ISUM) U1.18(VR_RDY) U1.19(VR_HOT_N) U1.21(RESET_N) U1.23(ENABLE) U1.24(PMB_CLK) U1.25(PMB_ALERT_N) U1.26(PMB_DIO) U1.27(VR_FAULT_N) U1.28(ADDR_TRISE) U1.29(SLEW-MODE) U1.30(O-USR) U1.31(VBOOT) U1.32(F-IMAX) U1.33(NC) U1.34(NC) U1.35(PWM4) U1.36(PWM3) U1.37(PWM2) U1.38(PWM1) U1.39(SKIP_NVM_N) U1.40(TSEN) V3V3.1(+) V3V3.2(-) V5.1(+) V5.2(-) VALERT.1 VIN.1(+) VIN.2(-) VSCL.1 VSDA.1

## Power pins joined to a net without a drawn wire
BOOT_R: M1.8(BOOT_R) M2.8(BOOT_R) M3.8(BOOT_R) M4.8(BOOT_R)
GND: U1.17(GND) U1.20(GND) U1.22(GND)
PAD: U1.41(PAD)
PGND: M1.4(PGND) M1.13(PGND) M2.4(PGND) M2.13(PGND) M3.4(PGND) M3.13(PGND) M4.4(PGND) M4.13(PGND)
V3R3: U1.14(V3R3)
V5: U1.15(V5)
V12: U1.16(V12)
VDD: M1.5(VDD) M2.5(VDD) M3.5(VDD) M4.5(VDD)
VIN: M1.7(VIN) M2.7(VIN) M3.7(VIN) M4.7(VIN)
VREF: U1.13(VREF)
VSW: M1.6(VSW) M2.6(VSW) M3.6(VSW) M4.6(VSW)

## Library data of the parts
_CSP1_1 _CSP1_2 _CSP2_1 _CSP2_2 _CSP3_1 _CSP3_2 _CSP4_1 _CSP4_2 _SKIP_1-_SKIP_5 _TSEN_1-_TSEN_5 _V3V3_1-_V3V3_5 _VREF_1-_VREF_6 _VRFAULT_1 _VRHOT_1 _VRRDY_1 _VSN_1 _VSN_2 _VSP_1 _VSP_2 = AcceleratedDesigns_Lib:WB_CONTINUATION; Manufacturer_Part_Number: WB_CONTINUATION
C3V3 CBP3 = AcceleratedDesigns_Lib:C0603C105Z8VACTU; Manufacturer_Part_Number: C0603C105Z8VACTU; Vendor: Kemet
CBST1-CBST4 = AcceleratedDesigns_Lib:EMK107B7104KA-T; Manufacturer_Part_Number: EMK107B7104KA-T; Vendor: Taiyo Yuden
CCOMP = AcceleratedDesigns_Lib:GRM1555C1H102JA01J; Manufacturer_Part_Number: GRM1555C1H102JA01J; Vendor: MuRata
CCOMP2 = AcceleratedDesigns_Lib:CL21C220JBANNNC; Manufacturer_Part_Number: CL21C220JBANNNC; Vendor: Samsung Electro-Mechanics
CDD = AcceleratedDesigns_Lib:C1608X5R1E105K080AC; Manufacturer_Part_Number: C1608X5R1E105K080AC; Vendor: TDK
CEN1-CEN4 CSNUB1-CSNUB4 = AcceleratedDesigns_Lib:CC0603JRNPO8BN102; Manufacturer_Part_Number: CC0603JRNPO8BN102; Vendor: Yageo America
CHF1-CHF4 = AcceleratedDesigns_Lib:CGA1A2X7R1E332K030BA; Manufacturer_Part_Number: CGA1A2X7R1E332K030BA; Vendor: TDK
CIMON = AcceleratedDesigns_Lib:GRM033R71A222KA01D; Manufacturer_Part_Number: GRM033R71A222KA01D; Vendor: MuRata
CIN CIN_2 = AcceleratedDesigns_Lib:16SVPG270M; Manufacturer_Part_Number: 16SVPG270M; Vendor: Panasonic
CINX_CH1-CINX_CH4 = AcceleratedDesigns_Lib:MSASE21GBB5226MTNA01; Manufacturer_Part_Number: MSASE21GBB5226MTNA01; Vendor: Taiyo Yuden
CINX_CH5-CINX_CH8 = AcceleratedDesigns_Lib:GRM32ER61C476KE15L; Manufacturer_Part_Number: GRM32ER61C476KE15L; Vendor: MuRata
COUT COUT_2-COUT_4 = AcceleratedDesigns_Lib:EEFGX0D471R; Manufacturer_Part_Number: EEFGX0D471R; Vendor: Panasonic
COUTX_CH1 COUTX_CH1_2-COUTX_CH1_12 COUTX_CH2 COUTX_CH2_2-COUTX_CH2_12 = AcceleratedDesigns_Lib:GRM32EC80J107ME20L; Manufacturer_Part_Number: GRM32EC80J107ME20L; Vendor: MuRata
CREF = AcceleratedDesigns_Lib:C0603C334K8RACTU; Manufacturer_Part_Number: C0603C334K8RACTU; Vendor: Kemet
CREF1-CREF4 = AcceleratedDesigns_Lib:08053C104KAT2A; Manufacturer_Part_Number: 08053C104KAT2A; Vendor: AVX
CTAO1-CTAO4 CTSEN = AcceleratedDesigns_Lib:GRM033R71C102KA01D; Manufacturer_Part_Number: GRM033R71C102KA01D; Vendor: MuRata
CV5 = AcceleratedDesigns_Lib:C1608X5R1C475K080AC; Manufacturer_Part_Number: C1608X5R1C475K080AC; Vendor: TDK
CVDD1-CVDD4 = AcceleratedDesigns_Lib:EMK212BJ225KG-T; Manufacturer_Part_Number: EMK212BJ225KG-T; Vendor: Taiyo Yuden
GND10 GND14 GND17 GND18 GND29 GND34 GND36 GND38 GND40 GND42 GND44 GND46 GND49 GND62 GND72 GND73 GND75 GND77 GND79 = AcceleratedDesigns_Lib:WB_GND; Manufacturer_Part_Number: WB_GND
GND35 GND47 GND48 GND63 GND64 GND66-GND68 GND70 GND74 GND76 GND78 GND83-GND91 = AcceleratedDesigns_Lib:WB_GND_SIGNAL; Manufacturer_Part_Number: WB_GND_SIGNAL
L1-L4 = AcceleratedDesigns_Lib:7443082022; Manufacturer_Part_Number: 7443082022; Vendor: Wurth Elektronik
M1-M4 = AcceleratedDesigns_Lib:CSD95372BQ5M; Manufacturer_Part_Number: CSD95372BQ5M
RADDR RMODE = AcceleratedDesigns_Lib:CRCW040216K5FKED; Manufacturer_Part_Number: CRCW040216K5FKED; Vendor: Vishay-Dale
RBST1-RBST4 RDD RSN RSNUB1-RSNUB4 RSP RV5 RVDD1-RVDD4 = AcceleratedDesigns_Lib:CRCW04021R00FKED; Manufacturer_Part_Number: CRCW04021R00FKED; Vendor: Vishay-Dale
RCOMP = AcceleratedDesigns_Lib:CRCW04023K83FKED; Manufacturer_Part_Number: CRCW04023K83FKED; Vendor: Vishay-Dale
REN1-REN4 = AcceleratedDesigns_Lib:RC0201FR-0710KL; Manufacturer_Part_Number: RC0201FR-0710KL; Vendor: Yageo America
RF = AcceleratedDesigns_Lib:RC0201FR-0723K7L; Manufacturer_Part_Number: RC0201FR-0723K7L; Vendor: Yageo America
RIMAX = AcceleratedDesigns_Lib:CRCW040226K1FKED; Manufacturer_Part_Number: CRCW040226K1FKED; Vendor: Vishay-Dale
RIMON = AcceleratedDesigns_Lib:CRCW040249K9FKED; Manufacturer_Part_Number: CRCW040249K9FKED
RISUM = AcceleratedDesigns_Lib:CRCW04022K55FKED; Manufacturer_Part_Number: CRCW04022K55FKED; Vendor: Vishay-Dale
RLOAD = AcceleratedDesigns_Lib:WB_LOAD_RESISTOR; Manufacturer_Part_Number: WB_LOAD_RESISTOR
RNVM ROCPR = AcceleratedDesigns_Lib:CRCW040220K0FKED; Manufacturer_Part_Number: CRCW040220K0FKED; Vendor: Vishay-Dale
ROSR = AcceleratedDesigns_Lib:CRCW0402150KFKED; Manufacturer_Part_Number: CRCW0402150KFKED; Vendor: Vishay-Dale
RRAMP = AcceleratedDesigns_Lib:CRCW04024K32FKED; Manufacturer_Part_Number: CRCW04024K32FKED; Vendor: Vishay-Dale
RSLEW RTRISE = AcceleratedDesigns_Lib:CRCW040224K3FKED; Manufacturer_Part_Number: CRCW040224K3FKED; Vendor: Vishay-Dale
RTSEN = AcceleratedDesigns_Lib:CRCW0402121KFKED; Manufacturer_Part_Number: CRCW0402121KFKED; Vendor: Vishay-Dale
RUSR = AcceleratedDesigns_Lib:CRCW04029K31FKED; Manufacturer_Part_Number: CRCW04029K31FKED; Vendor: Vishay-Dale
RVBOOTB = AcceleratedDesigns_Lib:CRCW040239K2FKED; Manufacturer_Part_Number: CRCW040239K2FKED; Vendor: Vishay-Dale
RVBOOTT = AcceleratedDesigns_Lib:CRCW040226K7FKED; Manufacturer_Part_Number: CRCW040226K7FKED; Vendor: Vishay-Dale
U1 = AcceleratedDesigns_Lib:TPS53647RTAR; Manufacturer_Part_Number: TPS53647RTAR
V3V3 V5 = AcceleratedDesigns_Lib:WB_PRIMITIVE_BATTERY; Manufacturer_Part_Number: WB_PRIMITIVE_BATTERY
VALERT = AcceleratedDesigns_Lib:WB_PMBUS_ALERT; Manufacturer_Part_Number: WB_PMBUS_ALERT
VIN = AcceleratedDesigns_Lib:WB_BATTERY; Manufacturer_Part_Number: WB_BATTERY
VSCL = AcceleratedDesigns_Lib:WB_I2C_SCL; Manufacturer_Part_Number: WB_I2C_SCL
VSDA = AcceleratedDesigns_Lib:WB_I2C_SDA; Manufacturer_Part_Number: WB_I2C_SDA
